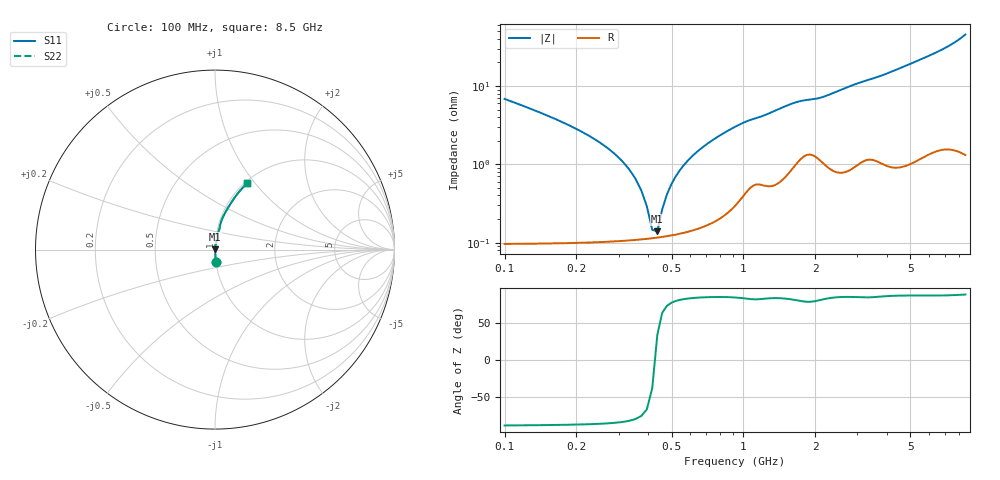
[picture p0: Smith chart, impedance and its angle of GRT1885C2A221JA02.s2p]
!Murata Part Number: GRT1885C2A221JA02
!These Parameters are Measured in Series Mode Connection
!Data Generated on Jun 19, 2026
!  o--ll--o
!Port1  Port2
!  o------o
!Operation Temp=25[degC], DC Bias Voltage=0[V]
!Freq. Start=100[MHz] Stop=9[GHz] 401[Steps]
# Hz S RI R 50
!Freq.(Hz) S11(Real) S11(Imag) S21(Real) S21(Imag) S12(Real) S12(Imag) S22(Real) S22(Imag)
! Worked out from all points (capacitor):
!   401 points, 100 MHz to 8.5 GHz, reference 50 ohm
!   read as one part in series: C = 220 pF near 142 MHz
!   lowest |Z| = 139 mohm at 436 MHz (marker M1)
!   series resonance near 426.4 MHz, so ESL is about 630 pH
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1e8  0.0056 -0.0679  0.9944 0.0679  0.9944 0.0679  0.0056 -0.0679
1.42e8  0.00302 -0.0451  0.997 0.0451  0.997 0.0451  0.00302 -0.0451
2.89e8  0.00122 -0.0135  0.9988 0.0135  0.9988 0.0135  0.00122 -0.0135
3.31e8  0.00114 -0.00869  0.9989 0.00869  0.9989 0.00869  0.00114 -0.00869
3.52e8  0.00112 -0.00655  0.9989 0.00655  0.9989 0.00655  0.00112 -0.00655
3.94e8  0.00112 -0.00269  0.9989 0.00269  0.9989 0.00269  0.00112 -0.00269
4.15e8  0.00114 -0.000914  0.9989 0.000914  0.9989 0.000914  0.00114 -0.000914
4.36e8  0.00116 0.000769  0.9988 -0.000769  0.9988 -0.000769  0.00116 0.000769
4.57e8  0.00119 0.00238  0.9988 -0.00238  0.9988 -0.00238  0.00119 0.00238
4.99e8  0.00126 0.00541  0.9987 -0.00541  0.9987 -0.00541  0.00126 0.00541
5.2e8  0.00131 0.00684  0.9987 -0.00684  0.9987 -0.00684  0.00131 0.00684
5.62e8  0.00142 0.00959  0.9986 -0.00959  0.9986 -0.00959  0.00142 0.00959
6.25e8  0.00164 0.0135  0.9984 -0.0135  0.9984 -0.0135  0.00164 0.0135
7.3e8  0.00213 0.0195  0.9979 -0.0195  0.9979 -0.0195  0.00213 0.0195
8.56e8  0.00307 0.0263  0.9969 -0.0263  0.9969 -0.0263  0.00307 0.0263
1.003e9  0.00512 0.0336  0.9949 -0.0336  0.9949 -0.0336  0.00512 0.0336
1.507e9  0.00994 0.0542  0.9901 -0.0542  0.9901 -0.0542  0.00994 0.0542
2.914e9  0.0195 0.1011  0.9805 -0.1011  0.9805 -0.1011  0.0195 0.1011
4.3e9  0.0327 0.1516  0.9673 -0.1516  0.9673 -0.1516  0.0327 0.1516
5.707e9  0.0599 0.2116  0.9401 -0.2116  0.9401 -0.2116  0.0599 0.2116
7.114e9  0.1016 0.2785  0.8984 -0.2785  0.8984 -0.2785  0.1016 0.2785
8.5e9  0.1784 0.3687  0.8216 -0.3687  0.8216 -0.3687  0.1784 0.3687
